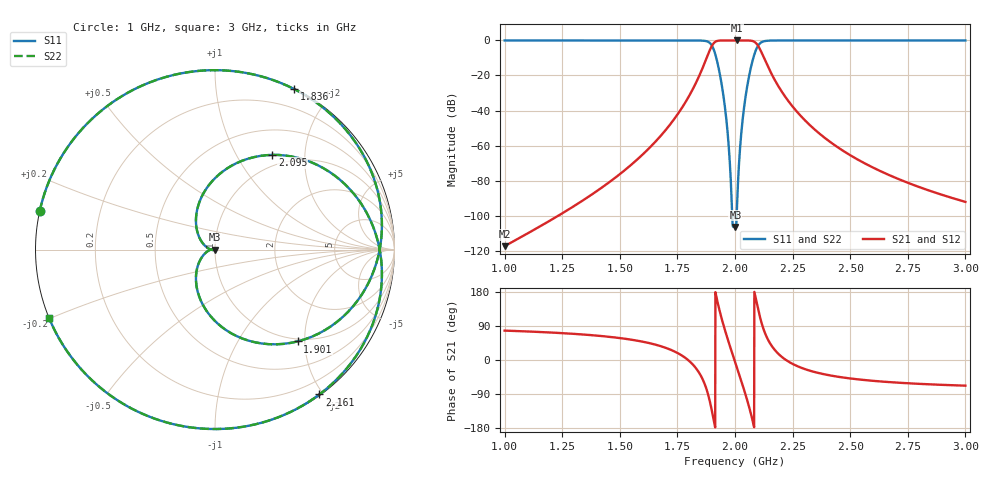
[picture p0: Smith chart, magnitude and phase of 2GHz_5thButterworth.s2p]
! Touchstone file from project
# GHZ S MA R 50.000000
! Modal data exported
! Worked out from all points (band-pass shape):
!   2001 points, 1 GHz to 3 GHz, reference 50 ohm
!   highest |S21| = 0.00 dB at 2.007 GHz (marker M1); lowest = -117.5 dB at 1 GHz (marker M2)
!   |S21| within 3 dB of the highest: 1.9 GHz to 2.1 GHz (199.9 MHz wide, 10 % of centre)
!   lowest |S11| = -106.5 dB at 2.002 GHz (marker M3), VSWR 1.00, Z = 50 + j5.6e-05 ohm
!   |S11| at or under -10 dB: 1.919 GHz to 2.079 GHz (160.6 MHz wide, 8.03 % of centre)
!   |S22| runs from -106.5 to 0.0 dB; largest |S21 - S12| = 0
!   S11 on the Smith chart (normalised r, x): 1 GHz: 0.00, +0.11; 1.836 GHz: 0.00, +1.60; 1.901 GHz: 0.95, -1.85; 2.095 GHz: 0.84, +1.42; 2.161 GHz: 0.01, -1.95; 3 GHz: 0.00, -0.20
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1  1 167.6  1.339e-06 77.6  1.339e-06 77.6  1 167.6
! Port Impedance 5.000000E+001 0.000000E+000 5.000000E+001 0.000000E+000
1.334  1 157.6  2.562e-05 67.6  2.562e-05 67.6  1 157.6
1.469  1 150.2  0.0001061 60.2  0.0001061 60.2  1 150.2
1.667  1 128.4  0.001581 38.4  0.001581 38.4  1 128.4
1.765  0.9999 103.5  0.0107 13.5  0.0107 13.5  0.9999 103.5
1.836  0.9973 63.9  0.0732 -26.1  0.0732 -26.1  0.9973 63.9
1.877  0.9479 11.8  0.3186 -78.2  0.3186 -78.2  0.9479 11.8
1.901  0.6882 -48.0  0.7255 -138.0  0.7255 -138.0  0.6882 -48.0
1.922  0.261 -111.1  0.9653 158.9  0.9653 158.9  0.261 -111.1
1.949  0.02853 -175.7  0.9996 94.3  0.9996 94.3  0.02853 -175.7
1.983  6.547e-05 121.2  1 27.1  1 27.1  6.547e-05 121.2
2  4.719e-06 174.8  1 -4.6  1 -4.6  4.719e-06 174.8
2.002  4.709e-06 173.2  1 -8.3  1 -8.3  4.709e-06 173.2
2.007  8.918e-06 -139.2  1 -17.6  1 -17.6  8.918e-06 -139.2
2.051  0.04102 168.0  0.9992 -102.0  0.9992 -102.0  0.04102 168.0
2.076  0.2615 111.0  0.9652 -159.0  0.9652 -159.0  0.2615 111.0
2.095  0.6166 58.8  0.7872 148.8  0.7872 148.8  0.6166 58.8
2.122  0.9323 -5.3  0.3617 84.7  0.3617 84.7  0.9323 -5.3
2.161  0.9947 -54.3  0.1032 35.7  0.1032 35.7  0.9947 -54.3
2.334  1 -119.8  0.003369 -29.8  0.003369 -29.8  1 -119.8
2.667  1 -148.2  0.0001454 -58.2  0.0001454 -58.2  1 -148.2
3  1 -157.8  2.464e-05 -67.8  2.464e-05 -67.8  1 -157.8
